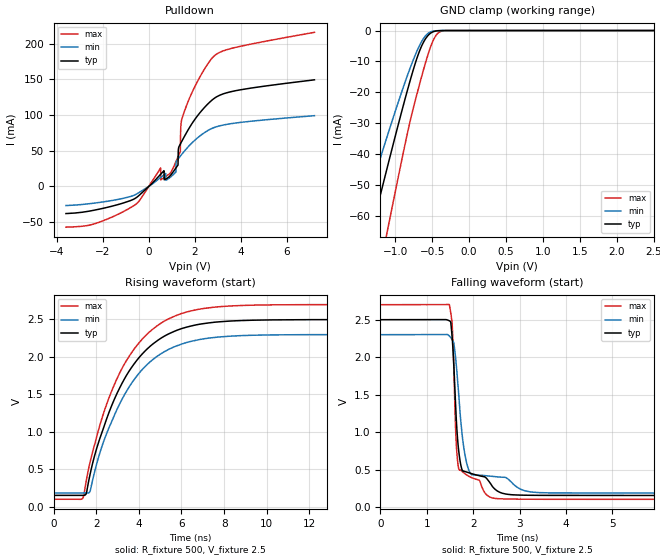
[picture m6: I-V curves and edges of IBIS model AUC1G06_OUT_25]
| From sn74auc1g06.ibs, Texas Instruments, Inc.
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[Model]   AUC1G06_OUT_25
Model_type  Open_drain
Enable   Active-Low
Vref =   0
Rref =   500
Cref =   30p
Vmeas =   1.25
| variable   typ   min   max
C_comp   2.81pF   2.34pF   3.34pF
| C_pulldown   3.33pF   0.95pF   5.35pF
| C_tri-state   2.81pF   2.34pF   3.34pF
[Temperature Range]   40   100   -40
| Ambient temperature   25   85   -40
[Voltage range]   2.5   2.3   2.7
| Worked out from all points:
|   slope of the pulldown table from 0 to 0.375 V, typ, clamps not added: 31 ohm
|   GND clamp passes 1 mA (typ) near -0.53 V on its own axis
|   rising waveform, R_fixture 500, V_fixture 2.5: 20-80 % time 2.26ns typ, 2.26ns min, 2.25ns max; typ from 0.154 V to 2.5 V
|   falling waveform, R_fixture 500, V_fixture 2.5: 20-80 % time 144ps typ, 213ps min, 97.3ps max; typ from 2.5 V to 0.154 V
[GND Clamp]
| AUC1G06_OUT_25
|   Voltage   I(typ)   I(min)   I(max)
-3.6V     -288.1mA   -237.2mA   -357.2mA
-1.505V   -82.55mA   -64.94mA   -112.2mA
-1.335V   -66.08mA   -51.59mA   -92.06mA
-1.28V    -60.78mA   -47.32mA   -85.53mA
-1.135V   -46.94mA   -36.23mA   -68.29mA
-1.09V    -42.69mA   -32.85mA   -62.95mA
-730mV    -10.76mA   -8.02mA    -22.8mA
-625mV    -4.167mA   -2.896mA   -13.43mA
-525mV    -931.1uA   -487.4uA   -5.581mA
-435mV    -114.4uA   -59.36uA   -1.201mA
-320mV    -4.035uA   -3.202uA   -34.93uA
2.5V      609.9pA    771.6pA    903.2pA
[Pulldown]
| AUC1G06_OUT_25
|   Voltage   I(typ)   I(min)   I(max)
-3.6V     -38.1mA    -26.84mA   -57.15mA
-1.13V    -23.5mA    -16.83mA   -35.77mA
515mV     17.02mA    12.57mA    25.99mA
520mV     17.2mA     12.7mA     9.298mA
930mV     15.07mA    12.68mA    18.6mA
1.27V     30.1mA     38.43mA    41.47mA
1.285V    51.84mA    39.04mA    42.6mA
1.37V     59.42mA    42.49mA    49.07mA
1.41V     61.85mA    44.1mA     90.07mA
1.65V     75.96mA    53.3mA     114.3mA
2.89V     124.5mA    83.17mA    184.3mA
7.2V      149.5mA    99.25mA    216.2mA
[Ramp]
| AUC1G06_OUT_25
| variable   typ   min   max
dV/dt_r   1.41/2.27E-09   1.27/2.26E-09   1.56/2.26E-09
dV/dt_f   1.41/1.46E-10   1.27/2.22E-10   1.56/9.98E-11
R_load = 500
[Rising Waveform]
| AUC1G06_OUT_25
R_fixture =   500
C_fixture =   0
L_fixture =   0
V_fixture =   2.5
V_fixture_min = 2.3
V_fixture_max = 2.7
|   Time   V(typ)   V(min)   V(max)
0s        154.5mV    186.3mV    102.6mV
1.375ns   154.4mV    186.2mV    117.2mV
1.535ns   178.4mV    186mV      348.1mV
1.72ns    442.7mV    216.7mV    604.8mV
2.25ns    977.2mV    790.2mV    1.163V
3.29ns    1.689V     1.477V     1.889V
4.55ns    2.148V     1.94V      2.346V
6.23ns    2.397V     2.192V     2.599V
10.23ns   2.494V     2.294V     2.695V
34.99ns   2.5V       2.3V       2.7V
[Falling Waveform]
| AUC1G06_OUT_25
R_fixture =   500
C_fixture =   0
L_fixture =   0
V_fixture =   2.5
V_fixture_min = 2.3
V_fixture_max = 2.7
|   Time   V(typ)   V(min)   V(max)
0s        2.5V       2.3V       2.7V
1.485ns   2.486V     2.283V     2.703V
1.545ns   2.271V     2.233V     2.456V
1.625ns   1.302V     1.962V     967.8mV
1.685ns   762.5mV    1.521V     517mV
1.79ns    478.5mV    821.4mV    459.2mV
1.915ns   455.5mV    476.4mV    407.4mV
2.475ns   234.2mV    404.9mV    114.8mV
3.645ns   155.3mV    188.7mV    103mV
34.99ns   154.5mV    186.3mV    102.6mV
